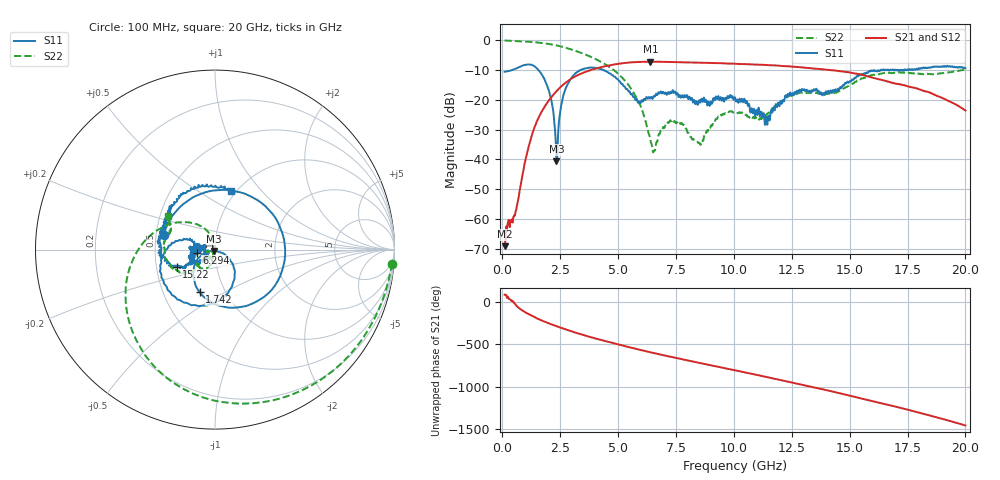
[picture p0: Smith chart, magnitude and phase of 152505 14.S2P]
!  2-Port S-parameters saved by WinCal
! VAR MeasName=S-Parameters (CALIBRATED_DATA) read from VNA (N5230C)
! VAR MeasDate=4/10/2015 9:29:40 AM
! VAR NAME=152505 14
! VAR FILENAME=152505 14.S2P
! VAR DATE=4/10/2015 9:29:40 AM
! VAR PHYS_PORTS=1,2
# Hz S DB R 50
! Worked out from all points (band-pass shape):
!   801 points, 100 MHz to 20 GHz, reference 50 ohm
!   highest |S21| = -7.20 dB at 6.393 GHz (marker M1); lowest = -69.2 dB at 100 MHz (marker M2)
!   |S21| within 3 dB of the highest: 3.748 GHz to 14.37 GHz (10.62 GHz wide, 117 % of centre)
!   lowest |S11| = -40.7 dB at 2.339 GHz (marker M3), VSWR 1.02, Z = 49.6 - j0.819 ohm
!   |S11| at or under -10 dB: start of sweep to 423.7 MHz; 1.561 GHz to 3.378 GHz (1.817 GHz wide, 73.6 % of centre); 4.376 GHz to 16.34 GHz (11.96 GHz wide, 115 % of centre)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
!   |S22| runs from -37.7 to -0.1 dB; largest |S21 - S12| = 0.0056
!   S11 on the Smith chart (normalised r, x): 100 MHz: 0.55, +0.10; 1.742 GHz: 0.76, -0.39; 6.294 GHz: 0.81, -0.03; 15.22 GHz: 0.64, -0.13; 20 GHz: 0.94, +0.70
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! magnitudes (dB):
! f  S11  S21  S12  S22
! 100 MHz  -10.6  -69.2  -68.1  -0.1
! 597.5 MHz  -9.5  -57.1  -57.1  -0.3
! 1.219 GHz  -8.2  -33.5  -33.5  -0.6
! 1.742 GHz  -12.0  -23.4  -23.4  -1.0
! 2.09 GHz  -19.2  -19.4  -19.4  -1.4
! 2.339 GHz  -40.7  -17.1  -17.1  -1.7
! 2.737 GHz  -16.2  -14.3  -14.3  -2.5
! 3.433 GHz  -9.8  -11.2  -11.1  -4.3
! 5.299 GHz  -15.7  -7.7  -7.7  -13.6
! 6.294 GHz  -19.6  -7.2  -7.2  -30.4
! 6.393 GHz  -19.6  -7.2  -7.2  -33.5
! 6.742 GHz  -17.5  -7.2  -7.2  -32.1
! 7.339 GHz  -17.1  -7.3  -7.3  -26.7
! 8.557 GHz  -20.9  -7.5  -7.5  -35.1
! 9.329 GHz  -18.7  -7.7  -7.7  -25.6
! 10.05 GHz  -19.2  -7.9  -7.9  -24.3
! 11.44 GHz  -28.4  -8.3  -8.3  -24.6
! 12.34 GHz  -18.0  -8.7  -8.8  -18.9
! 13.38 GHz  -17.1  -9.5  -9.4  -17.5
! 15.22 GHz  -12.6  -11.2  -11.1  -14.0
! 16.69 GHz  -10.1  -13.9  -14.0  -11.0
! 20 GHz  -9.4  -23.6  -23.6  -9.8
